(* Logix 5000 Rung export; software revision 16.04 *)

MODULES
   Local : vendor None type None code None
   MNET : vendor None type None code None
END_MODULES

TYPE MNETBLKSTAT :   // This object is used to store the block transfer statistics for the MVI56-MNET module.
STRUCT
   Read : INT;   // Total number of read block transfers
   Write : INT;   // Total number of write block transfers
   Parse : INT;   // Total number of blocks parsed
   Event : INT;   // Total number of event blocks received
   Cmd : INT;   // Total number of command blocks received
   Err : INT;   // Total number of block transfer errors
END_STRUCT
END_TYPE

TYPE MNETDATA :   // Contains Read Data (data read from the module to the processor) and Write Data (data written from the processor to the module)
STRUCT
   ReadData : INT[600];   // Data read from module. Set array equal to the size set in the Configuration file.
   WriteData : INT[600];   // Data to write to module. Set array equal to the size set in the Configuration file.
END_STRUCT
END_TYPE

TYPE MNETINITOUTDATA :   // Used to bring the Module into a known state after a restart operation.
STRUCT
   TriggerInitOut : BOOL;   // Trigger Output Data Initialization.
   InitializeOutputData : INT;   // Quantity of Blocks(200 words of "ReadData") for the module to read from the PLC. [0 to 24] means a qty of 1 to 25
   RetInitOutData : INT[200];   // Returned Initialization output data
   TriggerInitOutPending : BOOL;   // Set after the ladder has sent an event cmd to the module and is waiting for the status to be returned
   RetInitOutDataBlkID : INT;   // Returned Block ID for Returned Initialize Output Data command.
   InitOutBlkIDLim : INT;   // Block Index Limit for ReadData size of the array
END_STRUCT
END_TYPE

TYPE MNETUTIL :   // Variables for internal ladder usage - should not be accessed by user application
STRUCT
   CmdControl : MNETCMDCONTROL;   // Allows for a disabled command to be sent to a device(Server)
   EventCmd : MNETEVENTCMD;   // Event data to be used
   InitOutputData : MNETINITOUTDATA;   // This is to initialize output data module reads data from PLC
   PassThru : MNETPASSTHRU;   // This is to handle the pass thru format to be passed straight to the processor.
   IPsetPending : BOOL;   // Allows Setting module IP address
   IPgetPending : BOOL;   // Allows Getting module IP address
END_STRUCT
END_TYPE

TYPE MNETCONTROL :   // Values used by program for data transfer operation between the module and the processor.
STRUCT
   WarmBoot : BOOL;   // Causes software reset. The Module reads new configuration information.
   ColdBoot : BOOL;   // Causes hardware reset.
   BPLastRead : INT;   // Index of last read block
   BPLastWrite : INT;   // Index of last write block
   BlockIndex : INT;   // Computed block offset for data table
   WBPending : BOOL;   // Pending message
   CBPending : BOOL;   // Pending message
   ReadDataBlkCount : INT;   // Holds the value of the Block Counts of the Read Data Array. Array Size is divided by 200.
   WriteDataBlkCount : INT;   // Holds the value of the Block Counts of the Write Data Array. Array Size is divided by 200.
   RBTSremainder : INT;   // Holds remainder calculation value from the read array.
   WBTSremainder : INT;   // Holds remainder calculation value from the write array.
   ReadDataSizeGet : INT;   // Holds read data array size.
   WriteDataSizeGet : INT;   // Holds write data array size.
   IPAddress : MNETIPADDRESS;   // Getting and Setting IP address to and from Module
   FaultCode : INT;   // Fault Code value
   CheckInitialization : BOOL;   // Check Initialization trigger
END_STRUCT
END_TYPE

TYPE MNETPASSTHRU :   // Applicable with the selection of a Pass-Through mode (1 to 3) in the Configuration file.
STRUCT
   MBControl1 : CONTROL;   // Modbus pass thru message control
   MBControl2 : CONTROL;   // Modbus pass thru message control
   Mbdouble : DINT;   // Modbus double int tag
   MBMsg : SINT[500];   // Message array
   MBMsgLen : INT;   // Message length
   MBOffset : INT;   // Start offset in the message
   MBOffsetBit : INT;   // Offset bit in the message
   MBScratch : INT[3];   // Temporary used ints
   MBboolLength : DINT;   // Holds Word size that will accommodate Coil Qty.
   MBSpecial : INT[4];   // Holds Special Function 99 data.
   WriteDataDINTBuffer : DINT[50];   // Hold WriteData in DINT array
   InputDataDINTBuffer : DINT[50];   // Hold Connection Input Data in DINT array
END_STRUCT
END_TYPE

TYPE MNETMODULEDEF :   // This defines the whole module which includes all tags used in the program
STRUCT
   DATA : MNETDATA;   // Data read from module
   STATUS : MNETSTATUS;   // Client ,Server Status and blocks status
   CONTROL : MNETCONTROL;   // MNET Module control warmboot, coldboot, etc
   UTIL : MNETUTIL;   // command, event control
END_STRUCT
END_TYPE

TYPE MNETSTATUS :   // This status data is returned on each read block and can be used to detect proper module operation.
STRUCT
   PassCnt : INT;   // Program cycle counter
   ProductVersion : INT;   // Shows the module software version
   ProductCode : INT[2];   // This identifies the module product code
   MnetServStats : MNETSTATS;   // Server status for port 502
   MBAPServStats : MNETSTATS;   // Server status for port 2000
   ClientStats : MNETSTATS;   // Client Status
   BlockStats : MNETBLKSTAT;   // Block Transfer Statistics.
END_STRUCT
END_TYPE

TYPE MNETSTATS :   // This object is used to store the port statistics for an MVI56-MNET port.
STRUCT
   CmdReq : INT;   // Total number of command list requests sent
   CmdResp : INT;   // Total number of command list responses received
   CmdErr : INT;   // Total number of command list errors
   Requests : INT;   // Total number of requests for port
   Responses : INT;   // Total number of responses for port
   ErrSent : INT;   // Total number of errors sent
   ErrRec : INT;   // Total number of errors received
   CfgErrWord : INT;   // Configuration Error Word
   CurErr : INT;   // Current Error code
   LastErr : INT;   // Last recorded error code
END_STRUCT
END_TYPE

TYPE MNETCMDCONTROL :   // Controlling the Modbus Commands
STRUCT
   TriggerCmdCntrl : BOOL;   // Trigger Command Control. User application will activate this trigger.
   NumberOfCommands : INT;   // Number of commands per block (1 to 6)
   CommandIndex : INT[6];   // Stores the command indexes for command control.
   CmdsAddedToQueue : INT;   // Number of commands added to queue
   CmdControlBlockID : INT;   // Temporary variable to calculate control block ID
   CmdCntrlPending : BOOL;   // Auxiliary control command - prevents a second request before acknowledgment is received
END_STRUCT
END_TYPE

TYPE MNETIPADDRESS :   // Data structure to get and set the IP address of the module.
STRUCT
   IPGetTrigger : BOOL;   // Gets IP address.
   IPReceived : INT[4];   // IP address received.
   IPSetTrigger : BOOL;   // Sets IP address
   IPRequested : INT[4];   // IP address set.
END_STRUCT
END_TYPE

TYPE MNETEVENTCMD :   // Data structure to use for Event message generation.
STRUCT
   EventCmdTrigger : BOOL;   // Trigger for event command. User ladder must set this bit to initiate event command
   EventCmdPending : BOOL;   // Set after the ladder has sent an event cmd to the module and is waiting for the status to be returned
   IPAddress : INT[4];   // Server IP address. example: 192.168.0.101
   ServicePort : INT;   // TCP Service Port number (0-65535), 502 for MBAP, 2000 for MNET
   SlaveAddress : INT;   // Modbus slave NODE address (0 to 247)
   InternalDBAddress : INT;   // Internal database address
   PointCount : INT;   // Number of points for this command
   SwapCode : INT;   // Swap code (0= no swap, 1=swap words, 2=swap words and bytes, 3=swap bytes)
   ModbusFunctionCode : INT;   // Modbus function code
   DeviceDBAddress : INT;   // Target Server Modbus Address.
   EventCmdStatusReturned : INT;   // (0=Fail, 1=Success)
   EventBlockID : INT;   // Temporary variable to calculate event block ID
END_STRUCT
END_TYPE

ADD_ON_INSTRUCTION AOI56MNET   (* revision 1.61, vendor ProSoft Technology Inc., ExecutePrescan *)
// Add-On - MVI56-MNET and  MVI56E-MNET modules.
// Revision note:
// v1.61. resolves minor arithmetic overflow fault when msb of WriteData registers are set during a function 5 or 15 while passthru
VAR_IN_OUT
   Connection_Input : INT[250]; {required}   // Input parameters.
   Connection_Output : INT[248]; {required}   // Output parameters.
   MNET : MNETMODULEDEF; {required}
        .DATA.READDATA[0]   // Reads the RadData array size.
        ._UTIL.PASSTHRU.MBMSG[0]   // Modbus reserved. Always 0.
        ._UTIL.PASSTHRU.MBMSG[3]   // Modbus Function Code received.
        ._UTIL.PASSTHRU.MBOFFSET   // Starting Address for Modbus data set.
END_VAR
VAR
   MJFAULTS : DINT[12];
END_VAR

ROUTINE Logic   (* ladder *)
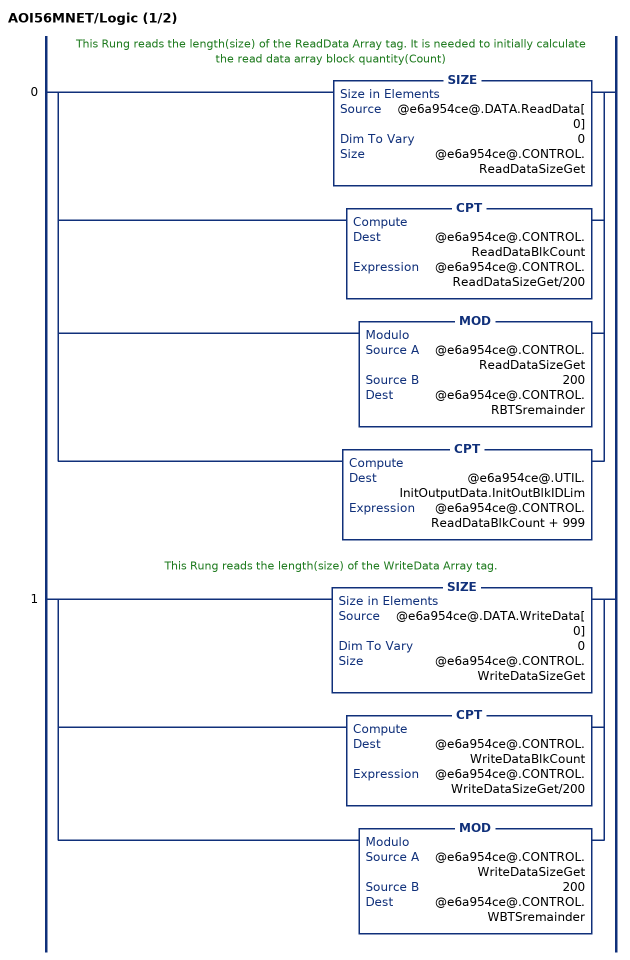
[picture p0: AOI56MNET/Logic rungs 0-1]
   // This Rung reads the length(size) of the ReadData Array tag. It is needed to initially calculate the read data array block quantity(Count)
   0: [SIZE(@e6a954ce@.DATA.ReadData[0],0,@e6a954ce@.CONTROL.ReadDataSizeGet) ,CPT(@e6a954ce@.CONTROL.ReadDataBlkCount,@e6a954ce@.CONTROL.ReadDataSizeGet/200) ,MOD(@e6a954ce@.CONTROL.ReadDataSizeGet,200,@e6a954ce@.CONTROL.RBTSremainder) ,CPT(@e6a954ce@.UTIL.InitOutputData.InitOutBlkIDLim,@e6a954ce@.CONTROL.ReadDataBlkCount + 999) ];
   // This Rung reads the length(size) of the WriteData Array tag.
   1: [SIZE(@e6a954ce@.DATA.WriteData[0],0,@e6a954ce@.CONTROL.WriteDataSizeGet) ,CPT(@e6a954ce@.CONTROL.WriteDataBlkCount,@e6a954ce@.CONTROL.WriteDataSizeGet/200) ,MOD(@e6a954ce@.CONTROL.WriteDataSizeGet,200,@e6a954ce@.CONTROL.WBTSremainder) ];
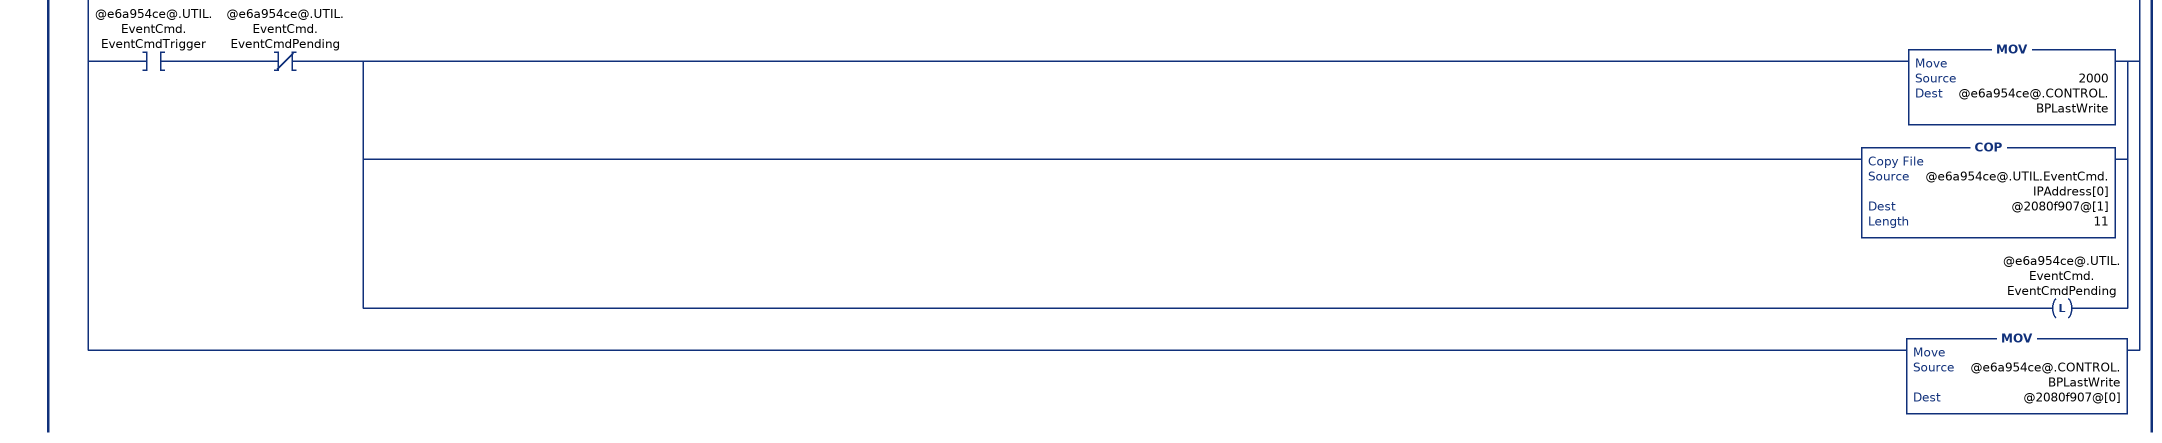
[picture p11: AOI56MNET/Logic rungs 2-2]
   // This rung is used to check for a new read block from the MVI56-MNET module in slot 1.  If new data is available, the LastRead and word[0] will not be equal.  This will force the program to call the ReadData subroutine to process the new data received.  After the new data is placed in the Modbus Data Table, the program will send new data to the module using the WriteData subroutine.
   2: NEQ(@7752de54@[249],@e6a954ce@.CONTROL.BPLastRead)[MOV(@7752de54@[249],@e6a954ce@.CONTROL.BPLastRead) ,GRT(@e6a954ce@.CONTROL.FaultCode,0) OTL(@e6a954ce@.CONTROL.CheckInitialization) ,EQU(@e6a954ce@.CONTROL.FaultCode,0) NEQ(@e6a954ce@.CONTROL.FaultCode,0) OTU(@e6a954ce@.CONTROL.CheckInitialization) ,EQU(@e6a954ce@.CONTROL.FaultCode,0) [EQU(-1,@e6a954ce@.CONTROL.BPLastRead) ,EQU(0,@e6a954ce@.CONTROL.BPLastRead) ] XIO(@e6a954ce@.CONTROL.CheckInitialization) [[EQU(@e6a954ce@.STATUS.ProductCode[1],13637) GEQ(@e6a954ce@.STATUS.ProductVersion,205) ,EQU(@e6a954ce@.STATUS.ProductCode[1],13652) GEQ(@e6a954ce@.STATUS.ProductVersion,151) ] [GEQ(@e6a954ce@.CONTROL.ReadDataSizeGet,200) COP(@7752de54@[2],@e6a954ce@.DATA.ReadData[0],200) ,LES(@e6a954ce@.CONTROL.ReadDataSizeGet,200) COP(@7752de54@[2],@e6a954ce@.DATA.ReadData[0],@e6a954ce@.CONTROL.RBTSremainder) ] ,COP(@7752de54@[202],@e6a954ce@.STATUS.PassCnt,1) ,COP(@7752de54@[203],@e6a954ce@.STATUS.BlockStats.Read,6) ,COP(@7752de54@[209],@e6a954ce@.STATUS.ProductCode[0],2) ,COP(@7752de54@[211],@e6a954ce@.STATUS.ProductVersion,1) ,COP(@7752de54@[219],@e6a954ce@.STATUS.MnetServStats.CmdReq,10) ,COP(@7752de54@[229],@e6a954ce@.STATUS.MBAPServStats.CmdReq,10) ,COP(@7752de54@[239],@e6a954ce@.STATUS.ClientStats.CmdReq,10) ] ,GEQ(@e6a954ce@.CONTROL.BPLastRead,1) [LEQ(@e6a954ce@.CONTROL.BPLastRead,@e6a954ce@.CONTROL.ReadDataBlkCount) [CPT(@e6a954ce@.CONTROL.BlockIndex,(@e6a954ce@.CONTROL.BPLastRead-1)*200) ,COP(@7752de54@[2],@e6a954ce@.DATA.ReadData[@e6a954ce@.CONTROL.BlockIndex],200) ] ,CMP(@e6a954ce@.CONTROL.BPLastRead - @e6a954ce@.CONTROL.ReadDataBlkCount = 1) GRT(@e6a954ce@.CONTROL.RBTSremainder,0) [CPT(@e6a954ce@.CONTROL.BlockIndex,(@e6a954ce@.CONTROL.BPLastRead-1)*200) ,COP(@7752de54@[2],@e6a954ce@.DATA.ReadData[@e6a954ce@.CONTROL.BlockIndex],@e6a954ce@.CONTROL.RBTSremainder) ] ,LEQ(@e6a954ce@.CONTROL.BPLastRead,25) [MOV(@7752de54@[202],@e6a954ce@.STATUS.PassCnt) ,COP(@7752de54@[203],@e6a954ce@.STATUS.BlockStats.Read,6) ,COP(@7752de54@[209],@e6a954ce@.STATUS.ProductCode[0],2) ,COP(@7752de54@[211],@e6a954ce@.STATUS.ProductVersion,1) ,COP(@7752de54@[219],@e6a954ce@.STATUS.MnetServStats.CmdReq,10) ,COP(@7752de54@[229],@e6a954ce@.STATUS.MBAPServStats.CmdReq,10) ,COP(@7752de54@[239],@e6a954ce@.STATUS.ClientStats.CmdReq,10) ] ] ,EQU(@e6a954ce@.CONTROL.BPLastRead,9990) [COP(@7752de54@[2],@e6a954ce@.CONTROL.IPAddress.IPRequested[0],4) ,OTU(@e6a954ce@.UTIL.IPsetPending) ] ,EQU(@e6a954ce@.CONTROL.BPLastRead,9991) [COP(@7752de54@[2],@e6a954ce@.CONTROL.IPAddress.IPReceived[0],4) ,OTU(@e6a954ce@.UTIL.IPgetPending) ] ,LIM(9956,@e6a954ce@.CONTROL.BPLastRead,9996) [EQU(9996,@e6a954ce@.CONTROL.BPLastRead) [MOV(@7752de54@[2],@e6a954ce@.UTIL.PassThru.MBMsgLen) ,COP(@7752de54@[3],@e6a954ce@.UTIL.PassThru.MBMsg[0],@e6a954ce@.UTIL.PassThru.MBMsgLen) ] ,LIM(9956,@e6a954ce@.CONTROL.BPLastRead,9957) [MOV(@7752de54@[3],@e6a954ce@.UTIL.PassThru.MBOffset) ,LES(@e6a954ce@.UTIL.PassThru.MBOffset,@e6a954ce@.CONTROL.WriteDataSizeGet) COP(@7752de54@[4],@e6a954ce@.DATA.WriteData[@e6a954ce@.UTIL.PassThru.MBOffset],@7752de54@[2]) ] ,EQU(9958,@e6a954ce@.CONTROL.BPLastRead) [MOV(@7752de54@[3],@e6a954ce@.UTIL.PassThru.MBOffsetBit) ,MOV(@7752de54@[4],@e6a954ce@.UTIL.PassThru.MBScratch[2]) ,DIV(@e6a954ce@.UTIL.PassThru.MBOffsetBit,16,@e6a954ce@.UTIL.PassThru.MBOffset) ,MOD(@e6a954ce@.UTIL.PassThru.MBOffsetBit,16,@e6a954ce@.UTIL.PassThru.MBOffsetBit) ,XPY(2,@e6a954ce@.UTIL.PassThru.MBOffsetBit,@e6a954ce@.UTIL.PassThru.mbdouble) ,MVM(@e6a954ce@.UTIL.PassThru.mbdouble,16#0000_ffff,@e6a954ce@.UTIL.PassThru.MBOffsetBit) ,COP(@e6a954ce@.DATA.WriteData[@e6a954ce@.UTIL.PassThru.MBOffset],@e6a954ce@.UTIL.PassThru.WriteDataDINTBuffer[0],1) ,GEQ(@e6a954ce@.UTIL.PassThru.MBOffset,0) LES(@e6a954ce@.UTIL.PassThru.MBOffset,@e6a954ce@.CONTROL.WriteDataSizeGet) LEQ(@e6a954ce@.UTIL.PassThru.MBOffset,2048) [NEQ(@e6a954ce@.UTIL.PassThru.MBScratch[2],0) OR(@e6a954ce@.UTIL.PassThru.MBOffsetBit,@e6a954ce@.DATA.WriteData[@e6a954ce@.UTIL.PassThru.MBOffset],@e6a954ce@.UTIL.PassThru.WriteDataDINTBuffer[0]) ,EQU(@e6a954ce@.UTIL.PassThru.MBScratch[2],0) [NOT(@e6a954ce@.UTIL.PassThru.MBOffsetBit,@e6a954ce@.UTIL.PassThru.MBOffsetBit) ,AND(@e6a954ce@.UTIL.PassThru.MBOffsetBit,@e6a954ce@.DATA.WriteData[@e6a954ce@.UTIL.PassThru.MBOffset],@e6a954ce@.UTIL.PassThru.WriteDataDINTBuffer[0]) ] ,COP(@e6a954ce@.UTIL.PassThru.WriteDataDINTBuffer[0],@e6a954ce@.DATA.WriteData[@e6a954ce@.UTIL.PassThru.MBOffset],1) ] ] ,EQU(9959,@e6a954ce@.CONTROL.BPLastRead) [[MOV(@7752de54@[3],@e6a954ce@.UTIL.PassThru.MBOffset) ,CPT(@e6a954ce@.UTIL.PassThru.MBControl1.LEN,@7752de54@[2]/2+(@7752de54@[2] MOD 2)) MOV(@e6a954ce@.UTIL.PassThru.MBControl1.LEN,@e6a954ce@.UTIL.PassThru.MBControl2.LEN) ,CPT(@e6a954ce@.UTIL.PassThru.MBboolLength,@e6a954ce@.UTIL.PassThru.MBOffset+@7752de54@[2]) ,COP(@7752de54@[4],@e6a954ce@.UTIL.PassThru.InputDataDINTBuffer[0],50) ,COP(@e6a954ce@.DATA.WriteData[@e6a954ce@.UTIL.PassThru.MBOffset],@e6a954ce@.UTIL.PassThru.WriteDataDINTBuffer[0],@e6a954ce@.UTIL.PassThru.MBControl1.LEN) ] ,LEQ(@e6a954ce@.UTIL.PassThru.MBboolLength,@e6a954ce@.CONTROL.WriteDataSizeGet) [FAL(@e6a954ce@.UTIL.PassThru.MBControl1,?,?,ALL,@e6a954ce@.UTIL.PassThru.WriteDataDINTBuffer[@e6a954ce@.UTIL.PassThru.MBControl1.POS],@e6a954ce@.UTIL.PassThru.WriteDataDINTBuffer[@e6a954ce@.UTIL.PassThru.MBControl1.POS] AND(NOT @e6a954ce@.UTIL.PassThru.InputDataDINTBuffer[25+@e6a954ce@.UTIL.PassThru.MBControl1.POS])) ,FAL(@e6a954ce@.UTIL.PassThru.MBControl2,?,?,ALL,@e6a954ce@.UTIL.PassThru.WriteDataDINTBuffer[@e6a954ce@.UTIL.PassThru.MBControl2.POS],@e6a954ce@.UTIL.PassThru.WriteDataDINTBuffer[@e6a954ce@.UTIL.PassThru.MBControl2.POS] OR(@e6a954ce@.UTIL.PassThru.InputDataDINTBuffer[25+@e6a954ce@.UTIL.PassThru.MBControl2.POS] AND @e6a954ce@.UTIL.PassThru.InputDataDINTBuffer[@e6a954ce@.UTIL.PassThru.MBControl2.POS])) ,RES(@e6a954ce@.UTIL.PassThru.MBControl1) ,RES(@e6a954ce@.UTIL.PassThru.MBControl2) ,COP(@e6a954ce@.UTIL.PassThru.WriteDataDINTBuffer[0],@e6a954ce@.DATA.WriteData[@e6a954ce@.UTIL.PassThru.MBOffset],@7752de54@[2]) ] ] ,LIM(9960,@e6a954ce@.CONTROL.BPLastRead,9961) [MOV(@7752de54@[3],@e6a954ce@.UTIL.PassThru.MBOffset) ,MOV(@7752de54@[2],@e6a954ce@.UTIL.PassThru.MBMsgLen) ,COP(@7752de54@[4],@e6a954ce@.DATA.WriteData[@e6a954ce@.UTIL.PassThru.MBOffset],@e6a954ce@.UTIL.PassThru.MBMsgLen) ,CPT(@e6a954ce@.UTIL.PassThru.MBMsgLen,@e6a954ce@.UTIL.PassThru.MBMsgLen*2+2) ,COP(@7752de54@[3],@e6a954ce@.UTIL.PassThru.MBMsg[0],@e6a954ce@.UTIL.PassThru.MBMsgLen) ] ,EQU(9970,@e6a954ce@.CONTROL.BPLastRead) COP(@2080f907@[0],@e6a954ce@.UTIL.PassThru.MBSpecial[0],4) ] ,LIM(5001,@e6a954ce@.CONTROL.BPLastRead,5006) [MOV(@e6a954ce@.CONTROL.BPLastRead,@e6a954ce@.UTIL.CmdControl.CmdControlBlockID) ,MOV(@7752de54@[2],@e6a954ce@.UTIL.CmdControl.CmdsAddedToQueue) ,OTU(@e6a954ce@.UTIL.CmdControl.CmdCntrlPending) ,OTU(@e6a954ce@.UTIL.CmdControl.TriggerCmdCntrl) ] ,EQU(@e6a954ce@.CONTROL.BPLastRead,2000) [MOV(@e6a954ce@.CONTROL.BPLastRead,@e6a954ce@.UTIL.EventCmd.EventBlockID) ,MOV(@7752de54@[2],@e6a954ce@.UTIL.EventCmd.EventCmdStatusReturned) ,OTU(@e6a954ce@.UTIL.EventCmd.EventCmdPending) ,OTU(@e6a954ce@.UTIL.EventCmd.EventCmdTrigger) ] ,MOV(@7752de54@[1],@e6a954ce@.CONTROL.BPLastWrite) ,XIC(@e6a954ce@.CONTROL.WarmBoot) [MOV(9998,@e6a954ce@.CONTROL.BPLastWrite) ,OTU(@e6a954ce@.CONTROL.WarmBoot) ] ,XIC(@e6a954ce@.CONTROL.ColdBoot) [MOV(9999,@e6a954ce@.CONTROL.BPLastWrite) ,OTU(@e6a954ce@.CONTROL.ColdBoot) ] ,[EQU(-1,@e6a954ce@.CONTROL.BPLastWrite) ,EQU(0,@e6a954ce@.CONTROL.BPLastWrite) ] [EQU(@e6a954ce@.STATUS.ProductCode[1],13637) GEQ(@e6a954ce@.STATUS.ProductVersion,205) ,EQU(@e6a954ce@.STATUS.ProductCode[1],13652) GEQ(@e6a954ce@.STATUS.ProductVersion,151) ] [GEQ(@e6a954ce@.CONTROL.WriteDataSizeGet,200) COP(@e6a954ce@.DATA.WriteData[0],@2080f907@[1],200) ,LES(@e6a954ce@.CONTROL.WriteDataSizeGet,200) COP(@e6a954ce@.DATA.WriteData[0],@2080f907@[1],@e6a954ce@.CONTROL.WBTSremainder) ] ,GEQ(@e6a954ce@.CONTROL.BPLastWrite,1) [LEQ(@e6a954ce@.CONTROL.BPLastWrite,@e6a954ce@.CONTROL.WriteDataBlkCount) [CPT(@e6a954ce@.CONTROL.BlockIndex,(@e6a954ce@.CONTROL.BPLastWrite-1)*200) ,COP(@e6a954ce@.DATA.WriteData[@e6a954ce@.CONTROL.BlockIndex],@2080f907@[1],200) ] ,CMP(@e6a954ce@.CONTROL.BPLastWrite - @e6a954ce@.CONTROL.WriteDataBlkCount = 1) GRT(@e6a954ce@.CONTROL.WBTSremainder,0) [CPT(@e6a954ce@.CONTROL.BlockIndex,(@e6a954ce@.CONTROL.BPLastWrite-1)*200) ,COP(@e6a954ce@.DATA.WriteData[@e6a954ce@.CONTROL.BlockIndex],@2080f907@[1],@e6a954ce@.CONTROL.WBTSremainder) ] ] ,LIM(1000,@e6a954ce@.CONTROL.BPLastWrite,1024) LEQ(@e6a954ce@.CONTROL.BPLastWrite,@e6a954ce@.UTIL.InitOutputData.InitOutBlkIDLim) [CPT(@e6a954ce@.CONTROL.BlockIndex,(@e6a954ce@.CONTROL.BPLastWrite-1000)*200) ,COP(@e6a954ce@.DATA.ReadData[@e6a954ce@.CONTROL.BlockIndex],@2080f907@[1],200) ] ,XIC(@e6a954ce@.CONTROL.IPAddress.IPSetTrigger) XIO(@e6a954ce@.UTIL.IPsetPending) [COP(@e6a954ce@.CONTROL.IPAddress.IPRequested[0],@2080f907@[1],4) ,MOV(9990,@e6a954ce@.CONTROL.BPLastWrite) ,OTU(@e6a954ce@.CONTROL.IPAddress.IPSetTrigger) ,OTL(@e6a954ce@.UTIL.IPsetPending) ] ,XIC(@e6a954ce@.CONTROL.IPAddress.IPGetTrigger) XIO(@e6a954ce@.UTIL.IPgetPending) [MOV(9991,@e6a954ce@.CONTROL.BPLastWrite) ,OTU(@e6a954ce@.CONTROL.IPAddress.IPGetTrigger) ,OTL(@e6a954ce@.UTIL.IPgetPending) ] ,XIC(@e6a954ce@.UTIL.CmdControl.TriggerCmdCntrl) XIO(@e6a954ce@.UTIL.CmdControl.CmdCntrlPending) [COP(@e6a954ce@.UTIL.CmdControl.CommandIndex[0],@2080f907@[1],6) ,LIM(1,@e6a954ce@.UTIL.CmdControl.NumberOfCommands,6) ADD(5000,@e6a954ce@.UTIL.CmdControl.NumberOfCommands,@e6a954ce@.CONTROL.BPLastWrite) ,OTL(@e6a954ce@.UTIL.CmdControl.CmdCntrlPending) ] ,XIC(@e6a954ce@.UTIL.EventCmd.EventCmdTrigger) XIO(@e6a954ce@.UTIL.EventCmd.EventCmdPending) [MOV(2000,@e6a954ce@.CONTROL.BPLastWrite) ,COP(@e6a954ce@.UTIL.EventCmd.IPAddress[0],@2080f907@[1],11) ,OTL(@e6a954ce@.UTIL.EventCmd.EventCmdPending) ] ,MOV(@e6a954ce@.CONTROL.BPLastWrite,@2080f907@[0]) ];
END_ROUTINE

ROUTINE Prescan   (* ladder *)
// Startup
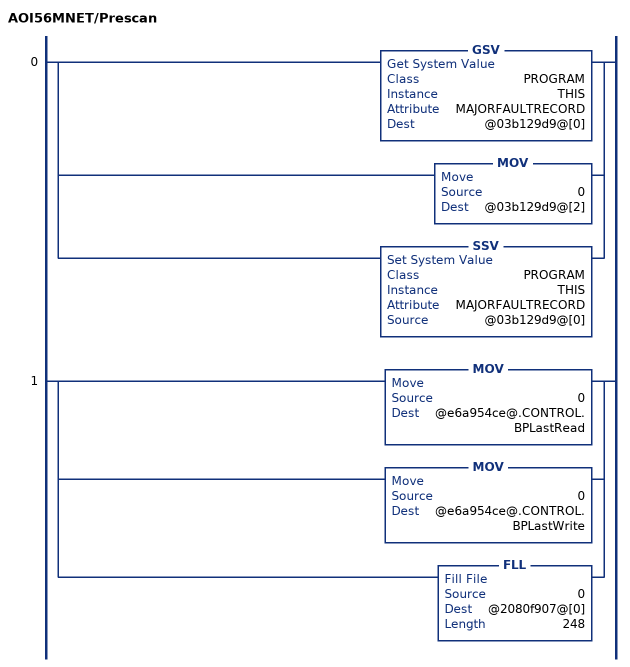
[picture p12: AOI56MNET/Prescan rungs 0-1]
   0: [GSV(PROGRAM,THIS,MAJORFAULTRECORD,@03b129d9@[0]) ,MOV(0,@03b129d9@[2]) ,SSV(PROGRAM,THIS,MAJORFAULTRECORD,@03b129d9@[0]) ];
   1: [MOV(0,@e6a954ce@.CONTROL.BPLastRead) ,MOV(0,@e6a954ce@.CONTROL.BPLastWrite) ,FLL(0,@2080f907@[0],248) ];
END_ROUTINE
END_ADD_ON_INSTRUCTION

VAR_GLOBAL   (* controller tags *)
   MNET : MNETMODULEDEF;   // Output parameters.
        .DATA.READDATA[0]   // Reads the ReadData array size.
        ._UTIL.PASSTHRU.MBMSG[0]   // Modbus reserved. Always 0.
        ._UTIL.PASSTHRU.MBMSG[3]   // Modbus Function Code received.
        ._UTIL.PASSTHRU.MBOFFSET   // Starting Address for Modbus data set.
   AOI56MNET : AOI56MNET;
   Local:2:I : AB:1756_MODULE_INT_500Bytes:I:0;
   Local:2:O : AB:1756_MODULE_INT_496Bytes:O:0;
END_VAR

PROGRAM MainProgram

ROUTINE MainRoutine   (* ladder *)
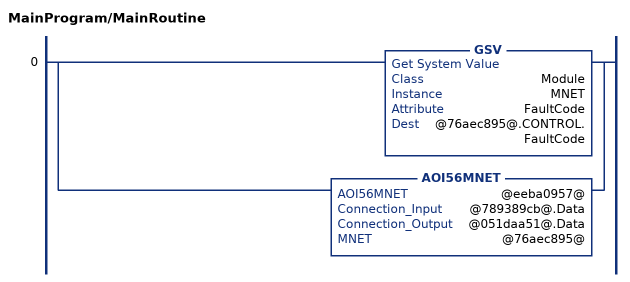
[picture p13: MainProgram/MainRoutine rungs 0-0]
   0: [GSV(Module,MNET,FaultCode,@76aec895@.CONTROL.FaultCode) ,AOI56MNET(@eeba0957@,@789389cb@.Data,@051daa51@.Data,@76aec895@) ];
END_ROUTINE
END_PROGRAM
